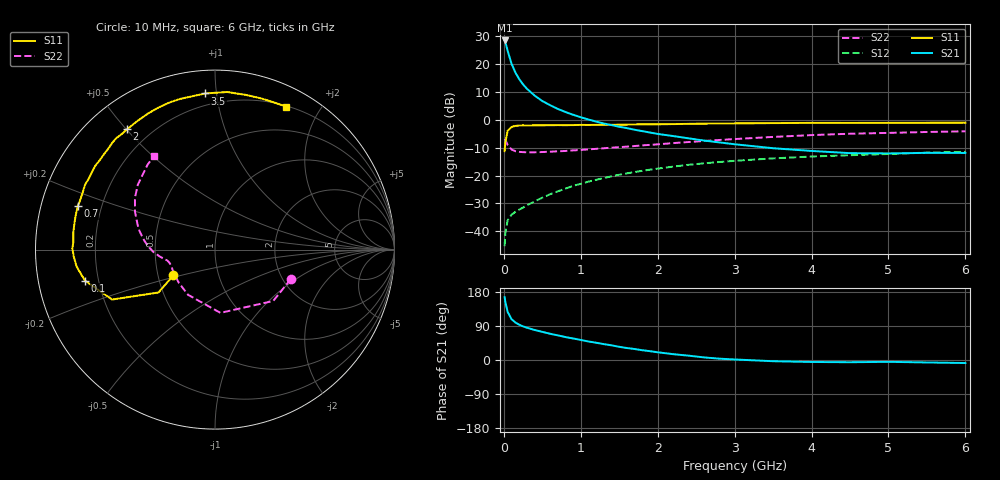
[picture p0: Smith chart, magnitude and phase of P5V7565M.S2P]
! SIEMENS Small Signal Semiconductors
! BFP183
! Si NPN RF Bipolar Junction Transistor in SOT143
! VCE = 0.75 V  IC = 65 mA
! Common Emitter S-Parameters:  March  1996
# GHz  S  MA  R  50
!  f  S11  S21  S12  S22
! GHz  MAG  ANG  MAG  ANG  MAG  ANG  MAG  ANG
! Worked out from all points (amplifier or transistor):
!   36 points, 10 MHz to 6 GHz, reference 50 ohm
!   highest |S21| = 28.5 dB at 10 MHz (marker M1)
!   |S21| within 3 dB of that: start of sweep to 42.7 MHz
!   unconditionally stable (mu >= 1): start of sweep to 45.76 MHz; 75.11 MHz to end of sweep
!   at 250 MHz: K = 1.61, MAG = 17.5 dB, |S12| = -31.5 dB
!   at 1.4 GHz: K = 2.16, MAG = 3.1 dB, |S12| = -20.3 dB
!   at 6 GHz: K = 1.52, MAG = -4.5 dB, |S12| = -11.5 dB
!   S11 on the Smith chart (normalised r, x): 10 MHz: 0.60, -0.19; 100 MHz: 0.15, -0.11; 700 MHz: 0.11, +0.15; 2 GHz: 0.12, +0.50; 3.5 GHz: 0.13, +0.93; 6 GHz: 0.21, +1.59
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0.01  0.2734 -148.2  26.5 165.9  0.0054 56.4  0.4534 -21.2
0.02  0.3952 -142.8  24.61 153.0  0.0094 54.9  0.4327 -41.4
0.05  0.6371 -154.1  17.2 126.6  0.0158 44.3  0.3538 -85.1
0.1  0.745 -166.6  10.12 107.8  0.0198 36.2  0.2932 -120.9
0.15  0.7769 -173.0  7.058 98.9  0.0223 38.2  0.2732 -137.7
0.2  0.7877 -177.1  5.351 93.1  0.0245 40.6  0.2658 -146.9
0.25  0.7949 179.5  4.31 88.7  0.0266 44.5  0.2629 -152.5
0.3  0.7903 177.0  3.609 85.2  0.0293 47.9  0.2609 -156.4
0.4  0.7954 172.9  2.719 79.2  0.0343 52.3  0.2612 -160.9
0.5  0.7971 169.0  2.171 74.3  0.04 54.9  0.2638 -163.7
0.6  0.7993 165.9  1.832 69.3  0.0461 56.9  0.268 -165.5
0.7  0.802 162.3  1.569 65.0  0.052 58.1  0.2716 -166.8
0.9  0.8033 156.6  1.231 56.8  0.0653 58.9  0.2821 -168.5
1.1  0.8067 150.7  1.011 48.9  0.0777 58.4  0.2947 -170.7
1.5  0.8154 139.6  0.75 34.8  0.1033 55.1  0.3226 -174.9
2  0.8303 126.1  0.557 20.4  0.133 49.2  0.3627 178.9
2.2  0.8367 121.3  0.511 15.4  0.1445 46.4  0.3816 175.5
2.8  0.8581 107.0  0.393 3.5  0.1746 38.1  0.4342 166.0
3.5  0.8717 93.6  0.309 -3.2  0.2029 28.8  0.493 154.7
4.5  0.8789 78.6  0.252 -5.9  0.2313 16.7  0.562 139.9
5.5  0.8836 68.0  0.255 -6.5  0.2577 6.6  0.604 128.5
6  0.8896 63.6  0.254 -8.0  0.2661 1.3  0.6214 123.3
